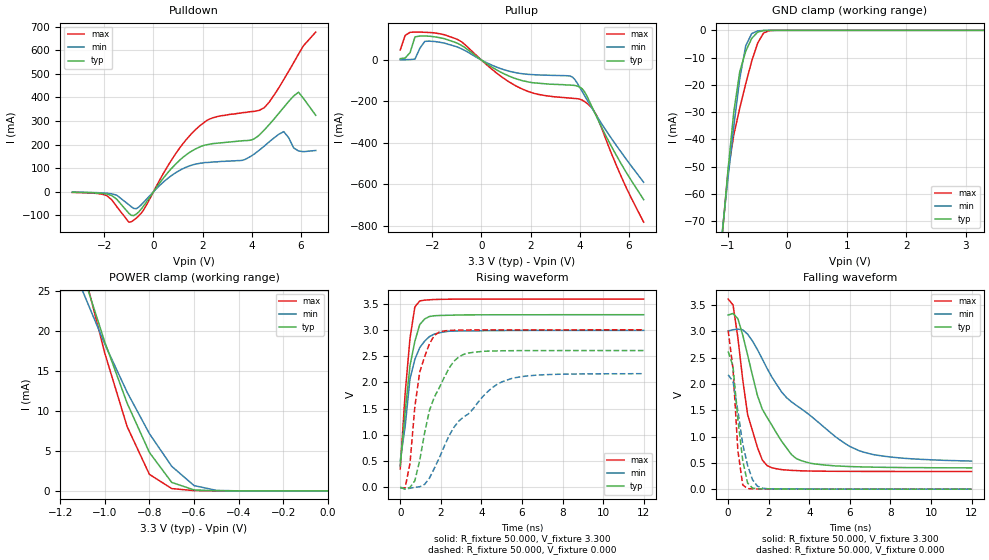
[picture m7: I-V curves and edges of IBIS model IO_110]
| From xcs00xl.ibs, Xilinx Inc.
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|   Model IO_110
[Model]   IO_110
Model_type   I/O
Polarity   Non-Inverting
Enable   Active-Low
Vinl =   0.800V
Vinh =   2.000V
Vmeas =   1.650V
Cref =  50.000pF
Rref =   1.000M
Vref =  0.000V
C_comp   5.300pF   3.500pF   6.800pF
[Temperature Range]   50.000   100.000   0.000
[Voltage Range]   3.300V   3.000V   3.600V
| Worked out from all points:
|   slope of the pulldown table from 0 to 0.495 V, typ, clamps not added: 7.07 ohm
|   slope of the pullup table from 0 to 0.495 V, typ, clamps not added: 12.6 ohm
|   GND clamp passes 1 mA (typ) near -0.52 V on its own axis
|   POWER clamp passes 1 mA (typ) near -0.69 V on its own axis
|   rising waveform, R_fixture 50.000, V_fixture 3.300: 20-80 % time 549ps typ, 596ps min, 413ps max; typ from 0.4 V to 3.3 V
|   rising waveform, R_fixture 50.000, V_fixture 0.000: 20-80 % time 1.19ns typ, 2.31ns min, 616ps max; typ from -0.013 V to 2.61 V
|   falling waveform, R_fixture 50.000, V_fixture 3.300: 20-80 % time 1.67ns typ, 3.56ns min, 842ps max; typ from 3.31 V to 0.405 V
|   falling waveform, R_fixture 50.000, V_fixture 0.000: 20-80 % time 432ps typ, 601ps min, 329ps max; typ from 2.62 V to 0 V
[Pulldown]
| voltage   I(typ)   I(min)   I(max)
-3.3V     -2.3mA     -1.8mA     -2.8mA
-1.9V     -9.7mA     -6.1mA     -16.3mA
-900mV    -100mA     -63.86mA   -127mA
-400mV    -59.92mA   -44.53mA   -76.62mA
700mV     94.99mA    66.07mA    129mA
1.6V      175mA      114mA      252mA
2.3V      202mA      125mA      309mA
3.6V      216mA      133mA      335mA
4.5V      261mA      193mA      356mA
5.3V      358mA      255mA      476mA
5.9V      422mA      173mA      584mA
6.6V      324mA      175mA      677mA
[Pullup]
| voltage   I(typ)   I(min)   I(max)
-3.3V     6.59mA     1.22mA     48.5mA
-3.1V     9.75mA     1.52mA     119mA
-2.7V     112mA      4.46mA     135mA
-2.3V     116mA      90.3mA     134mA
-1.7V     108mA      86.06mA    127mA
-800mV    69.91mA    53.59mA    87.42mA
1.6V      -97.48mA   -65.22mA   -137mA
3.6V      -121mA     -77.38mA   -184mA
4.2V      -154mA     -173mA     -201mA
4.7V      -278mA     -272mA     -271mA
5.7V      -505mA     -448mA     -567mA
6.6V      -675mA     -591mA     -784mA
[GND_clamp]
| voltage   I(typ)   I(min)   I(max)
-3.3V     -539mA     -461mA     -635mA
-1.1V     -76.29mA   -74.81mA   -76.3mA
-1V       -51.66mA   -54.6mA    -52.25mA
-900mV    -29.77mA   -35.09mA   -38.23mA
-800mV    -15.1mA    -17.65mA   -28.49mA
-700mV    -7.645mA   -5.66mA    -19.53mA
-600mV    -2.968mA   -1.205mA   -11.34mA
-500mV    -649uA     -202uA     -4.68mA
-400mV    -83.34uA   -28.89uA   -976uA
-300mV    -8.303uA   -3.567uA   -95.2uA
3.3V      90.24nA    487nA      4.544uA
[POWER_clamp]
| voltage   I(typ)   I(min)   I(max)
-3.3V     51.86mA    10.89mA    181mA
-3.1V     70.08mA    13.61mA    230mA
-3V       85.17mA    15.89mA    249mA
-2.9V     108mA      19.33mA    255mA
-2.8V     138mA      24.96mA    249mA
-1.1V     27.32mA    25.08mA    28.22mA
-1V       18.65mA    18.39mA    17.25mA
-900mV    11mA       12.37mA    8.069mA
-800mV    4.821mA    7.171mA    2.071mA
-700mV    1.064mA    3.083mA    296uA
-600mV    127uA      671uA      39.67uA
0V        90.25nA    23.31nA    5.636uA
[Ramp]
| variable   typ   min   max
dV/dt_r   1.567/1.192n   1.301/2.301n   1.805/0.602n
dV/dt_f   1.737/1.661n   1.479/3.552n   1.959/0.836n
R_load = 50.000
[Rising Waveform]
R_fixture = 50.000
V_fixture = 3.300
V_fixture_min = 3.000
V_fixture_max = 3.600
L_fixture = 0.000H
C_fixture = 0.000F
| time   V(typ)   V(min)   V(max)
0s        400mV      500mV      341mV
240ps     1.428V     1.148V     1.779V
480ps     2.319V     2.07V      2.843V
720ps     2.788V     2.442V     3.447V
960ps     3.108V     2.667V     3.563V
1.2ns     3.217V     2.791V     3.579V
1.44ns    3.265V     2.88V      3.585V
1.68ns    3.279V     2.928V     3.591V
2.4ns     3.289V     2.982V     3.596V
12ns      3.299V     2.999V     3.599V
[Rising Waveform]
R_fixture = 50.000
V_fixture = 0.000
V_fixture_min = 0.000
V_fixture_max = 0.000
L_fixture = 0.000H
C_fixture = 0.000F
| time   V(typ)   V(min)   V(max)
0s        -13.37mV   -9.16mV    -16.64mV
240ps     -43.22mV   -46.3mV    -22.03mV
480ps     -13.28mV   -28.53mV   446mV
720ps     115mV      -10.23mV   1.535V
960ps     505mV      -439uV     2.199V
1.44ns    1.464V     166mV      2.742V
1.92ns    1.895V     549mV      2.966V
2.88ns    2.487V     1.256V     3.004V
5.04ns    2.608V     2.016V     3.008V
12ns      2.612V     2.168V     3.009V
[Falling Waveform]
R_fixture = 50.000
V_fixture = 3.300
V_fixture_min = 3.000
V_fixture_max = 3.600
L_fixture = 0.000H
C_fixture = 0.000F
| time   V(typ)   V(min)   V(max)
0s        3.307V     3.004V     3.611V
240ps     3.338V     3.028V     3.5V
480ps     3.238V     3.039V     2.875V
960ps     2.547V     2.944V     1.416V
1.44ns    1.783V     2.653V     798mV
1.92ns    1.363V     2.293V     447mV
2.64ns    908mV      1.843V     371mV
3.36ns    581mV      1.592V     353mV
6.48ns    424mV      727mV      338mV
12ns      405mV      534mV      336mV
[Falling Waveform]
R_fixture = 50.000
V_fixture = 0.000
V_fixture_min = 0.000
V_fixture_max = 0.000
L_fixture = 0.000H
C_fixture = 0.000F
| time   V(typ)   V(min)   V(max)
0s        2.617V     2.172V     3.015V
240ps     2.33V      2.045V     2.28V
480ps     1.321V     1.483V     728mV
720ps     538mV      854mV      79.05mV
960ps     116mV      449mV      9.332mV
1.2ns     20.89mV    180mV      8.31mV
1.44ns    7.787mV    57.01mV    4.642mV
1.68ns    5.876mV    18.98mV    3.045mV
2.64ns    3.125mV    4.49mV     1.721mV
12ns      353uV      537uV      218uV
